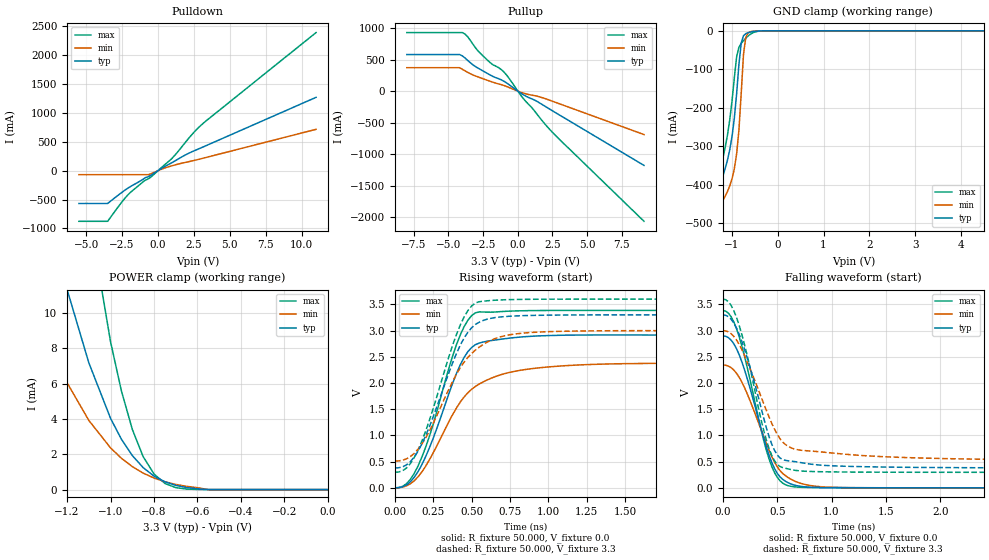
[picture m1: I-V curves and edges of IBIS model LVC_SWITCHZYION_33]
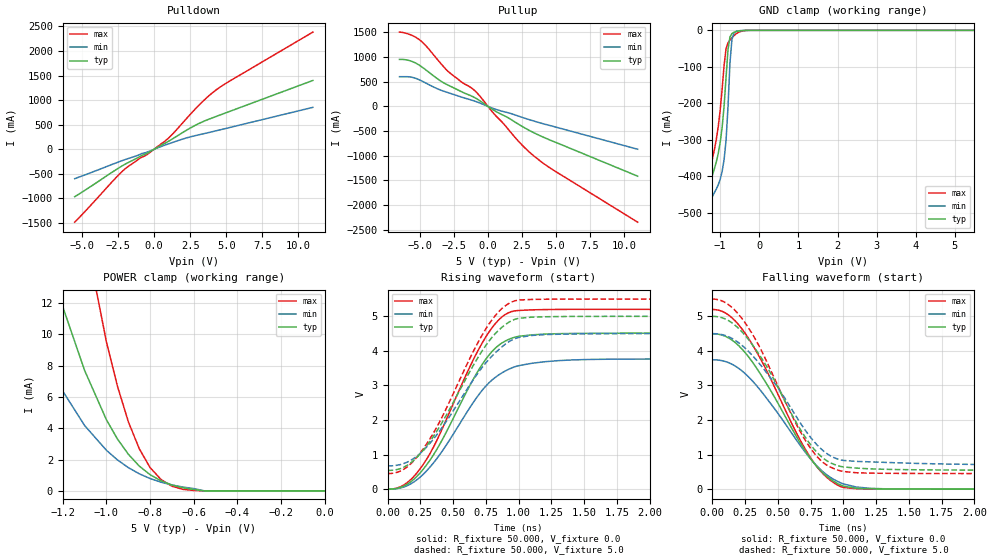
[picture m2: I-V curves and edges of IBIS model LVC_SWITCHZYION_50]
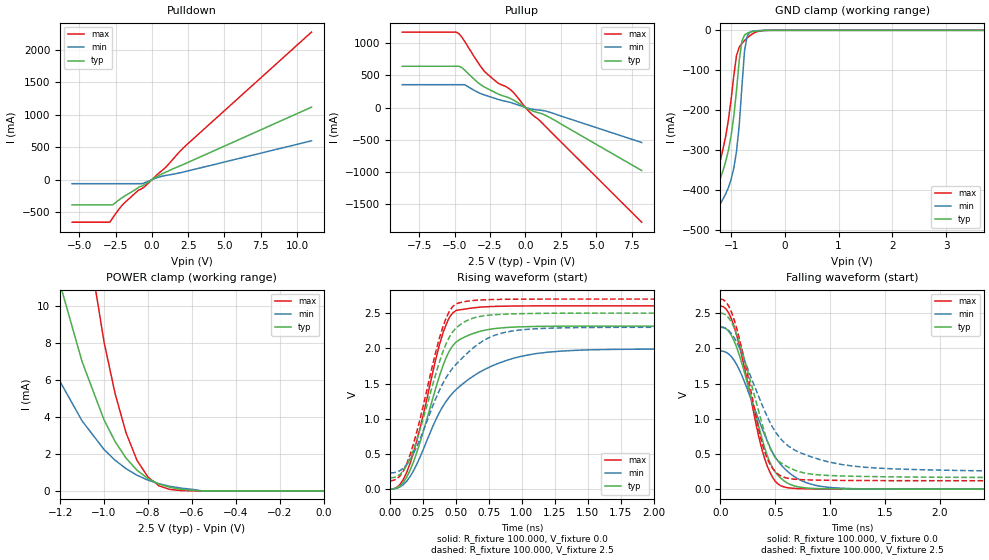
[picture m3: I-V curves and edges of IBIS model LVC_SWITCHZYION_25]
| Philips Semiconductors Inc.
| Logic Products Group
| IBIS model of 74LVC2G66
| 3.3V DUAL ANALOG SWITCH
|[Packages]:
|[Package1]: SOT505-2 (TSSOP) 8-Pin Package ;
|[Package2]: SOT765 (VSSOP) 8-Pin Package ;
[IBIS Ver]   3.2
[File Name]   lvc2g66.ibs
[File Rev]   1.0
[Date]   05-Aug-2003
[Source]   File created from simulations by LPG
   Philips Semiconductors Nijmegen
[Notes]   V1.0   Ibis model.
| Revision History
| Version Date   Author/ Description
|   Editor
| 1.0   August   2003 RM   Initial Version
| Remarks:
| 1. The Power Clamp curves have been omitted since there is no power clamp
|   diode.
| 2. Non-monotonic sections below 0V in pulldown and pullup curves have been
|   removed (if any).
[Disclaimer]
   (C) Copyright 2003 Philips Semiconductors
   All rights reserved
   Philips Semiconductors warrants and represents that the IBIS model
   identified herein is owned by Philips Semiconductors (PHILIPS). The
   model provided is not warranted as fully representing all of the
   operating characteristics and specifications of the semiconductor
   products to which the model relates.  Moreover, unless there is a
   signed, written agreement to the contrary, this IBIS model is
   furnished on an "as is" basis without support or warranty of any
   kind, either expressed or implied, regarding the use thereof, and
   PHILIPS specifically disclaims all implied warranties of
   merchantability and fitness of the model for any purpose.
   PHILIPS does not assume any liability arising out of the application
   or use of this IBIS model including infringement of patents and
   copyrights, nor does PHILIPS convey any license under its patents and
   copyrights or the rights of others.
   PHILIPS provides IBIS models as a service to our customers. You and
   your company shall not distribute, convey, sell, or give these models
   to anyone else without receiving prior written permission from
   PHILIPS.
   PHILIPS reserves the right to make changes without notice to these
   IBIS models to improve reliability, function, or design.
   Please be aware that your receipt and subsequent use of the IBIS
   information provided shall serve as acceptance of the terms and
   conditions of this agreement.  If you do not accept these terms,
   you should return or destroy the IBIS models and any other
   accompanying information immediately.
|   Info for  SOT505-2 (TSSOP) 8-Pin Package
[Component]   74LVC2G66_1
[Manufacturer]   Philips Semiconductors Inc.
[Package]
|   typ   min   max
R_pkg   5.4457E-02   4.6527E-02   6.2827E-02
L_pkg   1.399E-09   1.251E-09   1.584E-09
C_pkg   9.08E-14   7.40E-14   1.08E-13
[Pin] signal_name   model_name   R_pin   L_pin   C_pin
   1   Y1   lvc_switchzyion 6.28E-02 1.584E-09  1.08E-13
   2   Z1   lvc_switchyzion 4.72E-02 1.312E-09  7.50E-14
   3   E2   lvc_xgctrlin 4.65E-02 1.251E-09  7.40E-14
   4   GND   GND 6.15E-02 1.472E-09  1.07E-13
   5   Y2   lvc_switchzyion 6.22E-02 1.484E-09  1.07E-13
   6   Z2   lvc_switchyzion 4.69E-02 1.256E-09  7.40E-14
   7   E1   lvc_xgctrlin 4.67E-02 1.304E-09  7.40E-14
   8   VCC   POWER 6.18E-02 1.527E-09  1.07E-13
|   Info for  SOT765 (VSSOP) 8-Pin Package
[Component]   74LVC2G66_2
[Manufacturer]   Philips Semiconductors Inc.
[Package]
|   typ   min   max
R_pkg   3.2883E-02   1.0000E-06   4.2432E-02
L_pkg   9.425E-10   1.000E-12   1.184E-09
C_pkg   8.64E-14   1.00E-15   1.19E-13
[Pin] signal_name   model_name   R_pin   L_pin   C_pin
   1   Y1   lvc_switchzyion 4.24E-02 1.145E-09  1.19E-13
   2   Z1   lvc_switchyzion 3.40E-02 1.018E-09  8.30E-14
   3   E2   lvc_xgctrlin 3.40E-02 1.016E-09  8.40E-14
   4   GND   GND 4.24E-02  1.15E-09  1.19E-13
   5   Y2   lvc_switchzyion 3.40E-02  9.89E-10  1.12E-13
   6   Z2   lvc_switchyzion 3.40E-02 1.037E-09  8.30E-14
   7   E1   lvc_xgctrlin 4.24E-02 1.184E-09  9.00E-14
   8   VCC   POWER 1.00E-06  1.00E-12  1.00E-15
[Model Selector]   lvc_switchzyion
| Remark: If your software does not support the Model Selector
|   Please comment out the lines of the Model Selector, which
|   contain the name of the Model, except the one you want to use.
LVC_SWITCHZYION_33   3.3V-Vcc bilateral switch model
LVC_SWITCHZYION_50   5.0V-Vcc bilateral switch model
LVC_SWITCHZYION_25   2.5V-Vcc bilateral switch model
LVC_SWITCHZYION_18   1.8V-Vcc bilateral switch model
[Model Selector]   lvc_switchyzion
| Remark: If your software does not support the Model Selector
|   Please comment out the lines of the Model Selector, which
|   contain the name of the Model, except the one you want to use.
LVC_SWITCHYZION_33   3.3V-Vcc bilateral switch model
LVC_SWITCHYZION_50   5.0V-Vcc bilateral switch model
LVC_SWITCHYZION_25   2.5V-Vcc bilateral switch model
LVC_SWITCHYZION_18   1.8V-Vcc bilateral switch model
[Model Selector]   lvc_xgctrlin
| Remark: If your software does not support the Model Selector
|   Please comment out the lines of the Model Selector, which
|   contain the name of the Model, except the one you want to use.
LVC_XGCTRLIN_33   3.3V-Vcc input model
LVC_XGCTRLIN_50   5.0V-Vcc input model
LVC_XGCTRLIN_25   2.5V-Vcc input model
LVC_XGCTRLIN_18   1.8V-Vcc input model
|   Model LVC_SWITCHZY_33
[Model]   LVC_SWITCHZY_33
Model_type Series_switch
C_comp   7.55pF   5.38pF   10.52pF
|Ambient temperature: 25   85   -40
[Temperature Range]   35   95   -30
[Voltage Range]   3.3V   3.0V   3.6V
[Off]
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[On]
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|   Model LVC_SWITCHZY_50
[Model]   LVC_SWITCHZY_50
Model_type Series_switch
C_comp   7.63pF   4.23pF   10.52pF
|Ambient temperature: 25   85   -40
[Temperature Range]   50   105   -10
[Voltage Range]   5.0V   4.5V   5.5V
[Off]
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[On]
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|   Model LVC_SWITCHZY_25
[Model]   LVC_SWITCHZY_25
Model_type Series_switch
C_comp   7.63pF   3.93pF   10.52pF
|Ambient temperature: 25   85   -40
[Temperature Range]   30   90   -35
[Voltage Range]   2.5V   2.3V   2.7V
[Off]
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[On]
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|   Model LVC_SWITCHZY_18
[Model]   LVC_SWITCHZY_18
Model_type Series_switch
C_comp   7.87pF   4.23pF   10.52pF
|Ambient temperature: 25   85   -40
[Temperature Range]   25   85   -40
[Voltage Range]   1.8V   1.65V   1.95V
[Off]
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[On]
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|   Model LVC_SWITCHYZ_33
[Model]   LVC_SWITCHYZ_33
Model_type Series_switch
C_comp   7.68pF   5.51pF   10.52pF
|Ambient temperature: 25   85   -40
[Temperature Range]   35   95   -30
[Voltage Range]   3.3V   3.0V   3.6V
[Off]
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[On]
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|   Model LVC_SWITCHYZ_50
[Model]   LVC_SWITCHYZ_50
Model_type Series_switch
C_comp   7.71pF   4.34pF   10.52pF
|Ambient temperature: 25   85   -40
[Temperature Range]   50   105   -10
[Voltage Range]   5.0V   4.5V   5.5V
[Off]
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[On]
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|   Model LVC_SWITCHYZ_25
[Model]   LVC_SWITCHYZ_25
Model_type Series_switch
C_comp   7.87pF   4.15pF   10.52pF
|Ambient temperature: 25   85   -40
[Temperature Range]   30   90   -35
[Voltage Range]   2.5V   2.3V   2.7V
[Off]
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[On]
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|   Model LVC_SWITCHYZ_18
[Model]   LVC_SWITCHYZ_18
Model_type Series_switch
C_comp   8.21pF   4.64pF   10.52pF
|Ambient temperature: 25   85   -40
[Temperature Range]   25   85   -40
[Voltage Range]   1.8V   1.65V   1.95V
[Off]
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[On]
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| Models and submodels in the file (20): LVC_SWITCHZYION_33 (I/O), LVC_SWITCHZY_33 (Series_switch), LVC_SWITCHZYION_50 (I/O), LVC_SWITCHZY_50 (Series_switch), LVC_SWITCHZYION_25 (I/O), LVC_SWITCHZY_25 (Series_switch), LVC_SWITCHZYION_18 (I/O), LVC_SWITCHZY_18 (Series_switch), LVC_SWITCHYZION_33 (I/O), LVC_SWITCHYZ_33 (Series_switch), LVC_SWITCHYZION_50 (I/O), LVC_SWITCHYZ_50 (Series_switch), LVC_SWITCHYZION_25 (I/O), LVC_SWITCHYZ_25 (Series_switch), LVC_SWITCHYZION_18 (I/O), LVC_SWITCHYZ_18 (Series_switch), LVC_XGCTRLIN_33 (Input), LVC_XGCTRLIN_50 (Input), LVC_XGCTRLIN_25 (Input), LVC_XGCTRLIN_18 (Input)
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|   Model LVC_SWITCHZYION_33
[Model]   LVC_SWITCHZYION_33
Model_type   I/O
Polarity   Non-Inverting
Enable   Active-High
Vinl  =  0.8V
Vinh  =  2.0V
Vmeas =  1.5V
Cref  =  50.0pF
Rref  =  0.5k
Vref  =  0.0V
C_comp   7.55pF   5.38pF   10.52pF
[Model Spec]
| Note: The input and output voltage ratings may be exceeded if the input and
|   output current ratings are observed (please refer to the data sheet)
|   Subparameter   typ   min   max
| Thresholds
Vinh   2.0   2.0   2.0
Vinl   0.8   0.8   0.8
| Overshoot
S_overshoot_high   6.5   6.5   6.5   | Static overshoot
S_overshoot_low   -0.5   -0.5   -0.5
D_overshoot_high   7.2   7.2   7.2   | Dynamic overshoot
D_overshoot_low   -0.95   -0.9   -1.0
D_overshoot_time   3n   3n   3n
| Timing Thresholds
Vmeas   1.5   1.5   1.5
|Ambient temperature:   25   85   -40
[Temperature Range]   35   95   -30
[Voltage Range]   3.3V   3.0V   3.6V
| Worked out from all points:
|   slope of the pulldown table from 0 to 0.495 V, typ, clamps not added: 6.61 ohm
|   slope of the pullup table from 0 to 0.495 V, typ, clamps not added: 7.15 ohm
|   GND clamp passes 1 mA (typ) near -0.48 V on its own axis
|   POWER clamp passes 1 mA (typ) near -0.82 V on its own axis
|   rising waveform, R_fixture 50.000, V_fixture 0.0: 20-80 % time 224ps typ, 293ps min, 211ps max; typ from 0 V to 2.9 V
|   rising waveform, R_fixture 50.000, V_fixture 3.3: 20-80 % time 230ps typ, 270ps min, 219ps max; typ from 0.379 V to 3.3 V
|   falling waveform, R_fixture 50.000, V_fixture 0.0: 20-80 % time 244ps typ, 275ps min, 232ps max; typ from 2.9 V to 0 V
|   falling waveform, R_fixture 50.000, V_fixture 3.3: 20-80 % time 240ps typ, 300ps min, 222ps max; typ from 3.3 V to 0.379 V
|Process Range   nominal   slow   fast
[Pulldown]
| voltage   I(typ)   I(min)   I(max)
-5.5V     -567.8mA   -69.27mA   -876.1mA
-3.5V     -567.8mA   -69.27mA   -876.1mA
-2.7V     -410.6mA   -69.27mA   -603.3mA
-2.1V     -303.3mA   -69.27mA   -420.5mA
-950mV    -133.7mA   -69.27mA   -174.9mA
-650mV    -100.3mA   -67.2mA    -136.6mA
1V        143.1mA    86.85mA    219.3mA
2.5V      342.3mA    176.1mA    664.1mA
3.1V      406.5mA    213.4mA    810.2mA
11V       1.27A      716.1mA    2.391A
[Pullup]
| voltage   I(typ)   I(min)   I(max)
-8V       579.5mA    371mA      927.9mA
-4.2V     579.5mA    371mA      927.9mA
-4V       559mA      346.5mA    927.9mA
-3.8V     523.9mA    320.6mA    903.8mA
-3.2V     411.2mA    252.9mA    733.1mA
-2.8V     356.3mA    219.7mA    620.8mA
-2V       256.3mA    156.3mA    452.8mA
-1V       156.6mA    88.94mA    303.7mA
400mV     -57.65mA   -30.98mA   -118.2mA
1.4V      -164.4mA   -80.51mA   -369.2mA
2.6V      -325.2mA   -168.5mA   -676mA
9.1V      -1.177A    -688.4mA   -2.063A
[GND_clamp]
| voltage   I(typ)   I(min)   I(max)
-5.5V     -5.614A    -5.239A    -6.241A
-1.45V    -575.8mA   -631.6mA   -538.9mA
-1.4V     -528.6mA   -584.8mA   -491.2mA
-1.3V     -438mA     -495.3mA   -398.9mA
-1.05V    -309mA     -403.2mA   -231.2mA
-950mV    -227mA     -358.4mA   -121.6mA
-850mV    -87.2mA    -258.5mA   -42.87mA
-800mV    -31.72mA   -162.3mA   -32.87mA
-750mV    -12.79mA   -60.97mA   -25.51mA
-700mV    -7.379mA   -16.89mA   -19.05mA
-600mV    -3.195mA   -2.373mA   -8.867mA
5.5V      1.334nA    8.4nA      179.7pA
[POWER_clamp]
| voltage   I(typ)   I(min)   I(max)
-8V       6.216A     6.248A     6.248A
-1.4V     22.2mA     14.85mA    48.61mA
-1.3V     16.37mA    9.134mA    36.09mA
-1.2V     11.33mA    6.049mA    25.01mA
-1.1V     7.181mA    3.919mA    15.67mA
-1V       4.033mA    2.362mA    8.37mA
-950mV    2.853mA    1.774mA    5.585mA
-900mV    1.93mA     1.302mA    3.417mA
-850mV    1.245mA    934uA      1.866mA
-750mV    443.9uA    447uA      350.3uA
-550mV    0A         0A         0A
0V        0A         0A         0A
[Ramp]
| variable   typ   min   max
dV/dt_r   1.740V/223.834ps   1.419V/292.941ps   2.029V/210.725ps
dV/dt_f   1.753V/240.093ps   1.493V/299.605ps   1.982V/221.673ps
R_load = 50.000
[Rising Waveform]
R_fixture   = 50.000
V_fixture   = 0.0
V_fixture_min = 0.0
V_fixture_max = 0.0
| time   V(typ)   V(min)   V(max)
0s        0V         0V         0V
75ps      55.97mV    37.69mV    79.96mV
150ps     308.6mV    209.9mV    415.7mV
225ps     767.9mV    538.8mV    988.4mV
425ps     2.345V     1.634V     2.914V
500ps     2.679V     1.882V     3.287V
550ps     2.763V     1.982V     3.356V
850ps     2.884V     2.257V     3.379V
1.5ns     2.916V     2.369V     3.385V
8.8ns     2.9V       2.366V     3.381V
[Rising Waveform]
R_fixture   = 50.000
V_fixture   = 3.3
V_fixture_min = 3.0
V_fixture_max = 3.6
| time   V(typ)   V(min)   V(max)
0s        379mV      510.9mV    296.6mV
75ps      438.5mV    553.5mV    379.4mV
150ps     698.9mV    736.6mV    720.1mV
225ps     1.172V     1.088V     1.296V
425ps     2.719V     2.289V     3.103V
500ps     3.055V     2.564V     3.471V
550ps     3.162V     2.686V     3.551V
750ps     3.274V     2.921V     3.591V
1.2ns     3.298V     2.992V     3.6V
8.8ns     3.3V       3.001V     3.6V
[Falling Waveform]
R_fixture   = 50.000
V_fixture   = 0.0
V_fixture_min = 0.0
V_fixture_max = 0.0
| time   V(typ)   V(min)   V(max)
0s        2.898V     2.344V     3.381V
75ps      2.82V      2.294V     3.266V
150ps     2.538V     2.108V     2.88V
375ps     950.9mV    980.2mV    909.6mV
450ps     482.7mV    596.5mV    405.2mV
525ps     210mV      330.2mV    136.1mV
625ps     74.69mV    165.7mV    29.09mV
825ps     10.51mV    37.98mV    5.746mV
1.2ns     2.713mV    3.374mV    1.434mV
8.8ns     -3.513uV   -70.21uV   -23.32nV
[Falling Waveform]
R_fixture   = 50.000
V_fixture   = 3.3
V_fixture_min = 3.0
V_fixture_max = 3.6
| time   V(typ)   V(min)   V(max)
0s        3.3V       3V         3.6V
75ps      3.217V     2.942V     3.483V
150ps     2.927V     2.736V     3.097V
225ps     2.468V     2.397V     2.513V
375ps     1.334V     1.609V     1.099V
450ps     830.3mV    1.228V     615.7mV
525ps     571mV      937.7mV    407.2mV
650ps     503.7mV    745.5mV    339.1mV
2.4ns     383.3mV    545.2mV    296.6mV
8.8ns     379mV      511.1mV    296.6mV
|   Model LVC_SWITCHZYION_50
[Model]   LVC_SWITCHZYION_50
Model_type   I/O
Polarity   Non-Inverting
Enable   Active-High
Vinl  =  1.5V
Vinh  =  3.5V
Vmeas =  2.5V
Cref  =  50.0pF
Rref  =  0.5k
Vref  =  0.0V
C_comp   7.63pF   4.23pF   10.52pF
[Model Spec]
| Note: The input and output voltage ratings may be exceeded if the input and
|   output current ratings are observed (please refer to the data sheet)
|   Subparameter   typ   min   max
| Thresholds
Vinh   3.5   3.15   3.85
Vinl   1.5   1.35   1.65
| Overshoot
S_overshoot_high   6.5   6.5   6.5   | Static overshoot
S_overshoot_low   -0.5   -0.5   -0.5
D_overshoot_high   11.0   11.0   11.0   | Dynamic overshoot
D_overshoot_low   -0.95   -0.9   -1.0
D_overshoot_time   3n   3n   3n
| Timing Thresholds
Vmeas   2.5   2.25   2.75
|Ambient temperature:   25   85   -40
[Temperature Range]   50   105   -10
[Voltage Range]   5.0V   4.5V   5.5V
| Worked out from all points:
|   slope of the pulldown table from 0 to 0.75 V, typ, clamps not added: 6.16 ohm
|   slope of the pullup table from 0 to 0.75 V, typ, clamps not added: 5.86 ohm
|   GND clamp passes 1 mA (typ) near -0.45 V on its own axis
|   POWER clamp passes 1 mA (typ) near -0.80 V on its own axis
|   rising waveform, R_fixture 50.000, V_fixture 0.0: 20-80 % time 386ps typ, 407ps min, 387ps max; typ from 0 V to 4.5 V
|   rising waveform, R_fixture 50.000, V_fixture 5.0: 20-80 % time 408ps typ, 421ps min, 403ps max; typ from 0.542 V to 5 V
|   falling waveform, R_fixture 50.000, V_fixture 0.0: 20-80 % time 426ps typ, 442ps min, 419ps max; typ from 4.5 V to 0 V
|   falling waveform, R_fixture 50.000, V_fixture 5.0: 20-80 % time 403ps typ, 426ps min, 398ps max; typ from 5 V to 0.542 V
|Process Range   nominal   slow   fast
[Pulldown]
| voltage   I(typ)   I(min)   I(max)
-5.5V     -965.9mA   -598.5mA   -1.484A
-2.3V     -353.4mA   -240.5mA   -476.3mA
-1.9V     -286.4mA   -199.1mA   -372.4mA
-950mV    -141.5mA   -101.5mA   -176.3mA
-450mV    -75.83mA   -54.58mA   -100.2mA
900mV     145.7mA    99.79mA    201.5mA
1.3V      215.1mA    140.6mA    315mA
2.8V      479.4mA    274mA      803.5mA
4V        634.9mA    355.2mA    1.14A
5.2V      766.6mA    440.3mA    1.382A
11V       1.401A     853.1mA    2.385A
[Pullup]
| voltage   I(typ)   I(min)   I(max)
-6.5V     952.8mA    602.3mA    1.507A
-5.7V     923.7mA    597.1mA    1.455A
-4.9V     809.7mA    520.5mA    1.322A
-3.5V     520.1mA    332.9mA    882.1mA
-2.9V     428.1mA    276.5mA    701.5mA
-900mV    167.2mA    100.4mA    302.6mA
400mV     -72.56mA   -42.27mA   -135.7mA
1.2V      -189.4mA   -109mA     -367.5mA
2.2V      -353.4mA   -192.5mA   -693.8mA
3.4V      -537.7mA   -299.3mA   -1.011A
4.8V      -709.5mA   -405.7mA   -1.291A
11V       -1.415A    -868.6mA   -2.348A
[GND_clamp]
| voltage   I(typ)   I(min)   I(max)
-5.5V     -4.658A    -4.678A    -4.68A
-1.45V    -594.2mA   -644.9mA   -559mA
-1.35V    -500.6mA   -552.1mA   -464.3mA
-1.25V    -419.9mA   -473.8mA   -380.5mA
-1.05V    -338mA     -423.8mA   -264.6mA
-900mV    -207.6mA   -354.8mA   -95.83mA
-850mV    -129mA     -301.9mA   -50.47mA
-800mV    -53.03mA   -210.2mA   -34.13mA
-750mV    -18.36mA   -89.63mA   -26.27mA
-700mV    -8.85mA    -25.49mA   -20.09mA
-600mV    -3.699mA   -3.017mA   -10.25mA
5.5V      6.124nA    26.74nA    3.266nA
[POWER_clamp]
| voltage   I(typ)   I(min)   I(max)
-6.5V     4.731A     4.763A     4.744A
-1.4V     22.45mA    17.1mA     47.32mA
-1.3V     16.64mA    9.839mA    35.78mA
-1.2V     11.76mA    6.375mA    25.46mA
-1.1V     7.697mA    4.178mA    16.61mA
-1V       4.542mA    2.594mA    9.515mA
-950mV    3.326mA    1.986mA    6.708mA
-900mV    2.347mA    1.491mA    4.433mA
-850mV    1.592mA    1.097mA    2.702mA
-750mV    646uA      558.8uA    727.5uA
-600mV    94.84uA    149.6uA    30.63uA
0V        0A         0A         0A
[Ramp]
| variable   typ   min   max
dV/dt_r   2.698V/386.417ps   2.254V/407.048ps   3.119V/386.637ps
dV/dt_f   2.675V/402.858ps   2.296V/426.124ps   3.029V/397.682ps
R_load = 50.000
[Rising Waveform]
R_fixture   = 50.000
V_fixture   = 0.0
V_fixture_min = 0.0
V_fixture_max = 0.0
| time   V(typ)   V(min)   V(max)
0s        0V         0V         0V
125ps     91.79mV    63.99mV    123.3mV
250ps     477mV      352.7mV    597mV
400ps     1.309V     1.008V     1.603V
625ps     2.976V     2.341V     3.514V
750ps     3.76V      2.983V     4.405V
875ps     4.234V     3.369V     4.99V
975ps     4.401V     3.546V     5.16V
1.8ns     4.513V     3.763V     5.202V
8.8ns     4.497V     3.757V     5.199V
[Rising Waveform]
R_fixture   = 50.000
V_fixture   = 5.0
V_fixture_min = 4.5
V_fixture_max = 5.5
| time   V(typ)   V(min)   V(max)
0s        541.9mV    672.7mV    451.4mV
125ps     638.6mV    743mV      578.6mV
250ps     1.026V     1.039V     1.05V
400ps     1.826V     1.698V     1.968V
650ps     3.551V     3.142V     3.951V
750ps     4.159V     3.655V     4.637V
875ps     4.689V     4.124V     5.234V
1ns       4.943V     4.389V     5.472V
1.7ns     5V         4.498V     5.5V
8.8ns     5V         4.5V       5.5V
[Falling Waveform]
R_fixture   = 50.000
V_fixture   = 0.0
V_fixture_min = 0.0
V_fixture_max = 0.0
| time   V(typ)   V(min)   V(max)
0s        4.496V     3.744V     5.199V
100ps     4.421V     3.692V     5.097V
225ps     4.059V     3.426V     4.642V
375ps     3.283V     2.821V     3.719V
625ps     1.633V     1.513V     1.753V
750ps     883.2mV    875mV      905.4mV
875ps     365.2mV    408.8mV    337.1mV
1ns       88.06mV    151.2mV    49.02mV
1.5ns     3.833mV    4.367mV    1.894mV
8.8ns     -3.86uV    -60.63uV   -45.96nV
[Falling Waveform]
R_fixture   = 50.000
V_fixture   = 5.0
V_fixture_min = 4.5
V_fixture_max = 5.5
| time   V(typ)   V(min)   V(max)
0s        5V         4.5V       5.5V
125ps     4.873V     4.407V     5.333V
275ps     4.334V     3.989V     4.672V
425ps     3.484V     3.316V     3.607V
650ps     1.866V     2.043V     1.814V
775ps     1.165V     1.381V     1.052V
875ps     818.1mV    1.027V     692.1mV
1ns       643mV      830.9mV    510.4mV
2.7ns     543.8mV    693.3mV    451.2mV
8.8ns     541.9mV    672.7mV    451.4mV
|   Model LVC_SWITCHZYION_25
[Model]   LVC_SWITCHZYION_25
Model_type   I/O
Polarity   Non-Inverting
Enable   Active-High
Vinl  =  0.7V
Vinh  =  1.7V
Vmeas =  1.25V
Cref  =  30.0pF
Rref  =  0.5k
Vref  =  0.0V
C_comp   7.63pF   3.93pF   10.52pF
[Model Spec]
| Note: The input and output voltage ratings may be exceeded if the input and
|   output current ratings are observed (please refer to the data sheet)
|   Subparameter   typ   min   max
| Thresholds
Vinh   1.7   1.7   1.7
Vinl   0.7   0.7   0.7
| Overshoot
S_overshoot_high   6.5   6.5   6.5   | Static overshoot
S_overshoot_low   -0.5   -0.5   -0.5
D_overshoot_high   7.2   7.2   7.2   | Dynamic overshoot
D_overshoot_low   -0.95   -0.9   -1.0
D_overshoot_time   3n   3n   3n
| Timing Thresholds
Vmeas   1.25   1.15   1.35
|Ambient temperature:   25   85   -40
[Temperature Range]   30   90   -35
[Voltage Range]   2.5V   2.3V   2.7V
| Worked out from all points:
|   slope of the pulldown table from 0 to 0.375 V, typ, clamps not added: 7.27 ohm
|   slope of the pullup table from 0 to 0.375 V, typ, clamps not added: 8.98 ohm
|   GND clamp passes 1 mA (typ) near -0.49 V on its own axis
|   POWER clamp passes 1 mA (typ) near -0.84 V on its own axis
|   rising waveform, R_fixture 100.000, V_fixture 0.0: 20-80 % time 229ps typ, 402ps min, 202ps max; typ from 0 V to 2.31 V
|   rising waveform, R_fixture 100.000, V_fixture 2.5: 20-80 % time 228ps typ, 350ps min, 204ps max; typ from 0.162 V to 2.5 V
|   falling waveform, R_fixture 100.000, V_fixture 0.0: 20-80 % time 247ps typ, 321ps min, 221ps max; typ from 2.31 V to 0 V
|   falling waveform, R_fixture 100.000, V_fixture 2.5: 20-80 % time 256ps typ, 388ps min, 218ps max; typ from 2.5 V to 0.162 V
|Process Range   nominal   slow   fast
[Pulldown]
| voltage   I(typ)   I(min)   I(max)
-5.5V     -389.1mA   -62.48mA   -655.1mA
-2.9V     -389.1mA   -62.48mA   -655.1mA
-2.7V     -389.1mA   -62.48mA   -588.4mA
-2.3V     -317.8mA   -62.48mA   -462.4mA
-1.9V     -255.6mA   -62.48mA   -358.6mA
-950mV    -123.9mA   -62.48mA   -167.6mA
-650mV    -93.57mA   -60.4mA    -132.2mA
700mV     88.79mA    51.99mA    141mA
1V        119.6mA    65.7mA     201.1mA
2.2V      236.3mA    118.2mA    495.4mA
11V       1.115A     597mA      2.27A
[Pullup]
| voltage   I(typ)   I(min)   I(max)
-8.7V     642.1mA    355.2mA    1.174A
-4.9V     642.1mA    355.2mA    1.174A
-4.7V     642.1mA    355.2mA    1.149A
-4.3V     584.3mA    355.2mA    1.032A
-3.5V     416mA      252.8mA    749mA
-2.9V     319.3mA    196mA      563.9mA
-1.9V     207.6mA    124.4mA    374.9mA
-1.3V     161.6mA    91.26mA    315.1mA
-900mV    122.2mA    67.38mA    245.8mA
200mV     -23.87mA   -12.38mA   -50.99mA
1.8V      -166.2mA   -79.59mA   -380.5mA
8.2V      -980.6mA   -544.6mA   -1.785A
[GND_clamp]
| voltage   I(typ)   I(min)   I(max)
-5.5V     -5.58A     -5.208A    -6.231A
-1.4V     -522.4mA   -578.3mA   -486.2mA
-1.35V    -476.1mA   -532.3mA   -439.2mA
-1.3V     -431.8mA   -488.7mA   -393.9mA
-1.05V    -299.4mA   -393mA     -223mA
-900mV    -149.5mA   -302.6mA   -62.97mA
-850mV    -75.51mA   -237.8mA   -42.15mA
-800mV    -26.99mA   -141.1mA   -32.74mA
-750mV    -11.67mA   -49.95mA   -25.32mA
-700mV    -7.036mA   -13.78mA   -18.77mA
-600mV    -3.031mA   -2.133mA   -8.504mA
5.5V      735.6pA    6.552nA    73.18pA
[POWER_clamp]
| voltage   I(typ)   I(min)   I(max)
-8.7V     6.914A     6.943A     6.957A
-1.4V     22.12mA    14.01mA    48.88mA
-1.3V     16.23mA    8.854mA    36.1mA
-1.2V     11.14mA    5.889mA    24.83mA
-1.1V     6.97mA     3.777mA    15.36mA
-1V       3.833mA    2.235mA    8.034mA
-950mV    2.672mA    1.659mA    5.268mA
-900mV    1.774mA    1.201mA    3.142mA
-850mV    1.118mA    847.3uA    1.656mA
-800mV    667.6uA    583.4uA    746.9uA
-650mV    92.02uA    153.8uA    20.31uA
0V        0A         0A         0A
[Ramp]
| variable   typ   min   max
dV/dt_r   1.385V/229.455ps   1.188V/402.006ps   1.561V/201.990ps
dV/dt_f   1.403V/256.385ps   1.241V/388.264ps   1.548V/218.036ps
R_load = 100.000
[Rising Waveform]
R_fixture   = 100.000
V_fixture   = 0.0
V_fixture_min = 0.0
V_fixture_max = 0.0
| time   V(typ)   V(min)   V(max)
0s        0V         -205.6fV   0V
75ps      48.32mV    32.23mV    69.79mV
125ps     171.7mV    113.9mV    239.3mV
200ps     513mV      347.7mV    677.9mV
400ps     1.754V     1.178V     2.216V
450ps     1.967V     1.313V     2.441V
525ps     2.122V     1.456V     2.547V
925ps     2.3V       1.853V     2.601V
1.5ns     2.316V     1.978V     2.603V
8.8ns     2.309V     1.981V     2.601V
[Rising Waveform]
R_fixture   = 100.000
V_fixture   = 2.5
V_fixture_min = 2.3
V_fixture_max = 2.7
| time   V(typ)   V(min)   V(max)
0s        161.6mV    230.5mV    119.7mV
75ps      211.4mV    264.7mV    190.6mV
150ps     434.7mV    417.5mV    487.8mV
350ps     1.665V     1.307V     1.984V
425ps     2.07V      1.588V     2.434V
475ps     2.237V     1.722V     2.596V
575ps     2.388V     1.913V     2.667V
825ps     2.482V     2.205V     2.695V
1.3ns     2.499V     2.291V     2.7V
8.8ns     2.5V       2.301V     2.7V
[Falling Waveform]
R_fixture   = 100.000
V_fixture   = 0.0
V_fixture_min = 0.0
V_fixture_max = 0.0
| time   V(typ)   V(min)   V(max)
0s        2.307V     1.963V     2.601V
75ps      2.243V     1.92V      2.505V
150ps     2.007V     1.765V     2.177V
350ps     888.6mV    985.6mV    742.4mV
425ps     485.9mV    691.6mV    335.7mV
500ps     242.8mV    455.5mV    111.1mV
600ps     96.67mV    269.2mV    24.26mV
825ps     11.99mV    71.16mV    4.577mV
1.2ns     2.493mV    7.49mV     1.455mV
8.8ns     -4.149uV   -70.38uV   -27.19nV
[Falling Waveform]
R_fixture   = 100.000
V_fixture   = 2.5
V_fixture_min = 2.3
V_fixture_max = 2.7
| time   V(typ)   V(min)   V(max)
0s        2.5V       2.3V       2.7V
75ps      2.433V     2.253V     2.603V
150ps     2.193V     2.085V     2.277V
350ps     1.099V     1.311V     841.3mV
425ps     693.1mV    1.036V     440.5mV
500ps     446.5mV    816.7mV    247.2mV
625ps     306.4mV    605.9mV    151.3mV
1.1ns     187.6mV    351.2mV    124.5mV
1.7ns     172.7mV    281.9mV    120.6mV
8.8ns     161.6mV    231mV      119.7mV
